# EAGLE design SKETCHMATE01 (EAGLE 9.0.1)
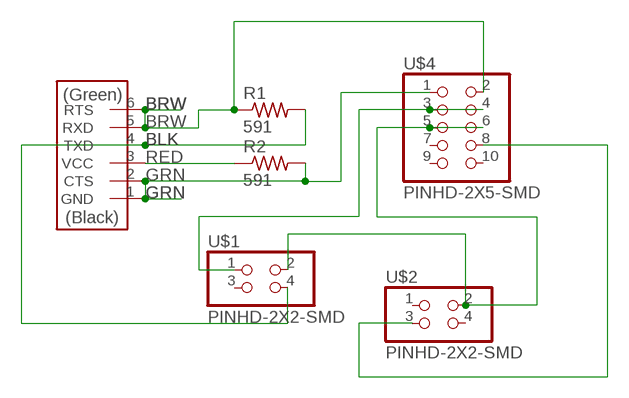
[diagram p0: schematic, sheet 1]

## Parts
R1  591  RES-US1206FAB  [R1206FAB]
R2  591  RES-US1206FAB  [R1206FAB]
U$1  PINHD-2X2-SMD  [2X02SMD]
U$2  PINHD-2X2-SMD  [2X02SMD]
U$4  PINHD-2X5-SMD  [2X05SMD]
YEL  FTDI-SMD-HEADER  [1X06SMD]

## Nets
BLK: R1.2 U$1.4 YEL.4(TXD)
BRW: R1.1 U$4.2 YEL.5(RXD) YEL.6(RTS)
GRN: R2.2 U$4.1 YEL.1(GND) YEL.2(CTS)
N$1: U$1.1 U$4.3 U$4.4
N$2: U$1.2 U$2.2 U$4.5 U$4.6
N$3: U$2.3 U$4.8
RED: R2.1 YEL.3(VCC)
Unconnected: U$1.3 U$2.1 U$2.4 U$4.7 U$4.9 U$4.10

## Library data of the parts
R1 R2 = fablibrary:RES-US: Resistor (US Symbol)
U$1 U$2 = fablibrary:PINHD-2X2-SMD
U$4 = fablibrary:PINHD-2X5-SMD
YEL = fablibrary:FTDI-SMD-HEADER

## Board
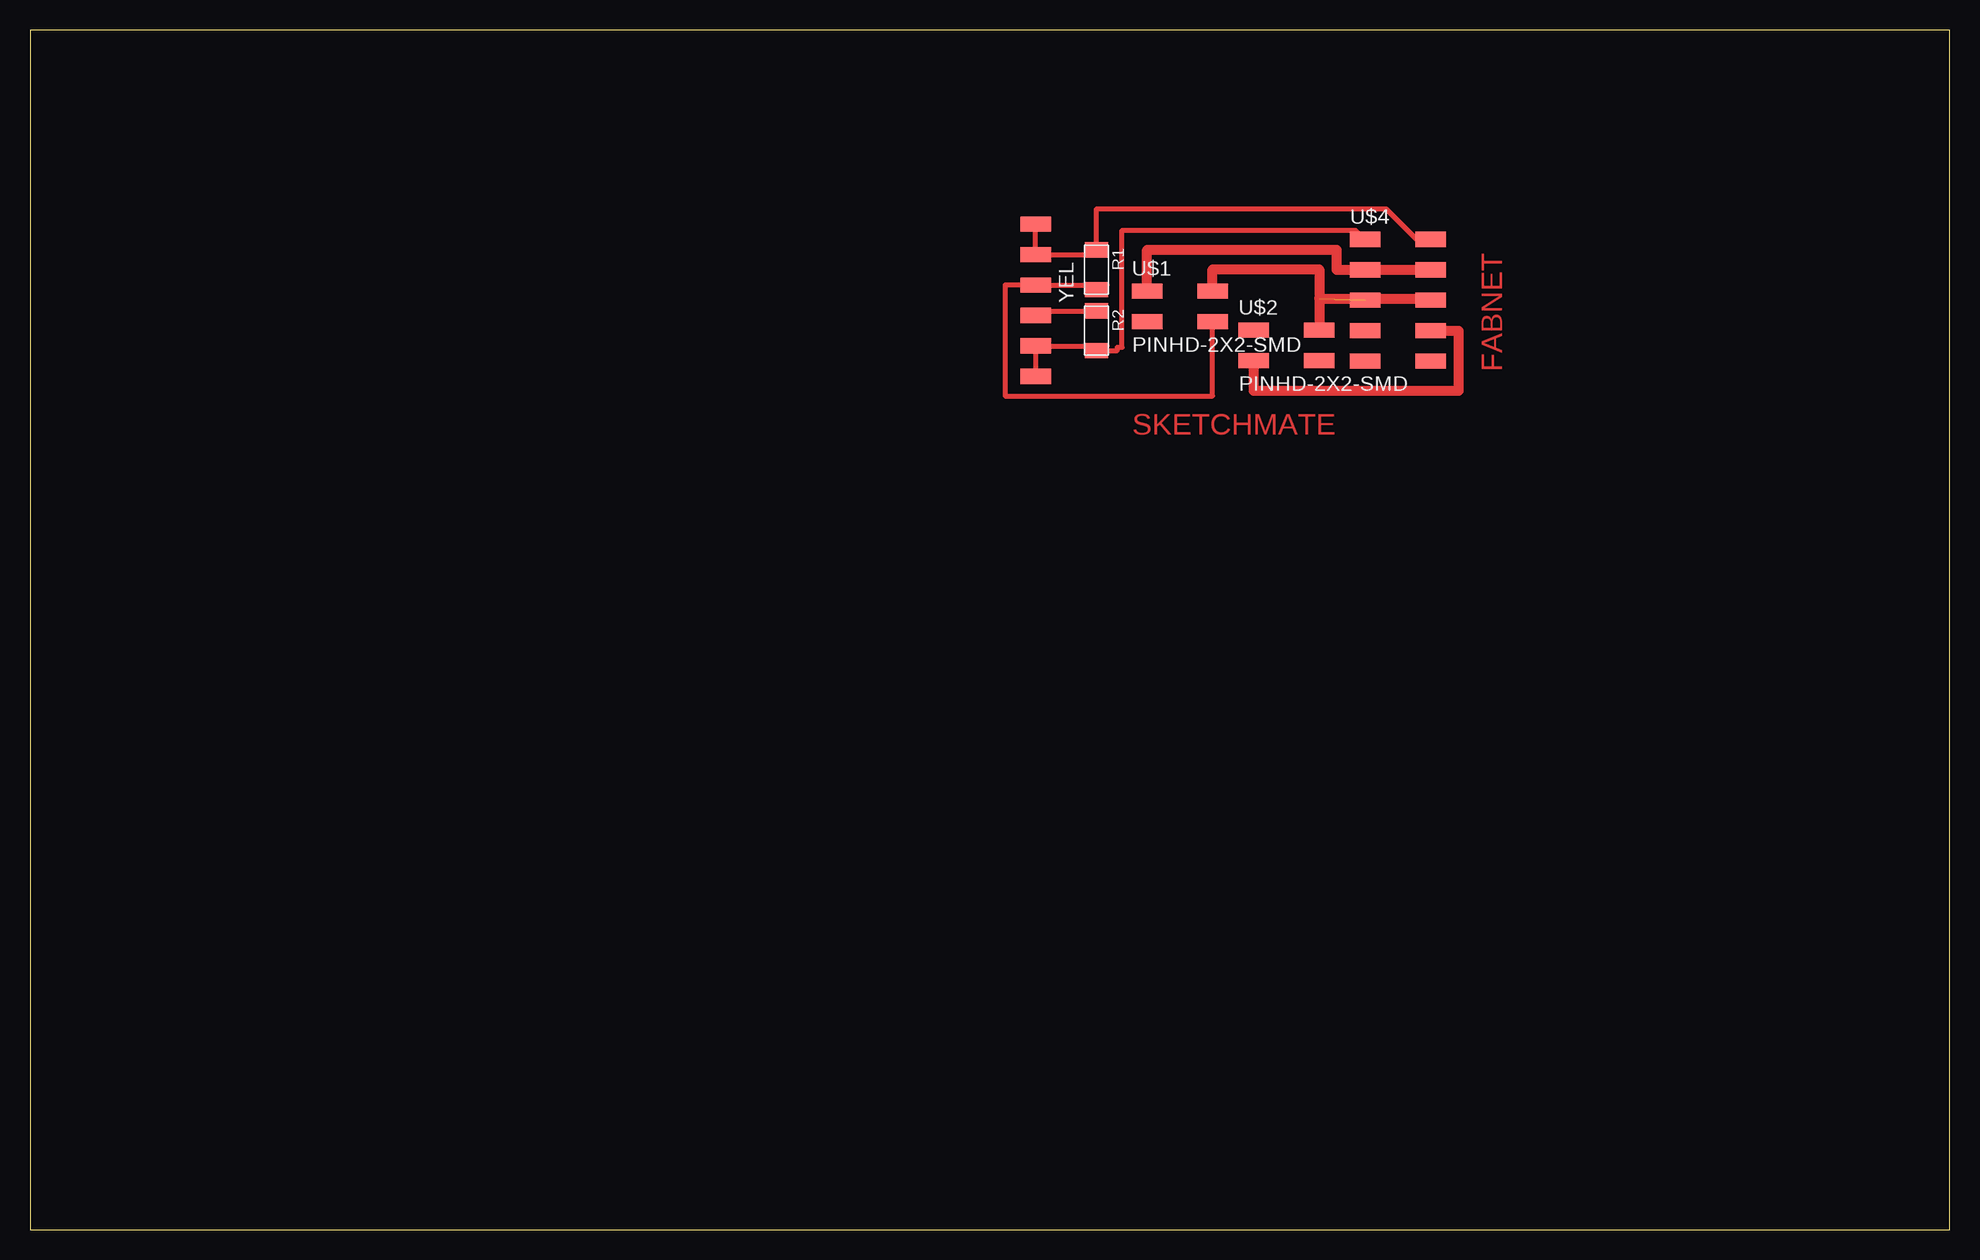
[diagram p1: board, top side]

Size 160 x 100 mm. Coordinates in mm from the lower left corner, seen from the top.
Outline: 0,0 160,0 160,100 0,100 0,0
Copper layers (1*16): Top 0.035mm / dielectric 1.5mm / Bottom 0.035mm
Design rules "default": minimum track width 6mil, minimum drill 0.35mm, track to track 6mil, track to pad 6mil, pad to pad 6mil, via to via 6mil, smd to smd 6mil, copper to edge 40mil, drill to drill 6mil, minimum pad ring 10mil, minimum via ring 8mil, stop-mask expansion 4mil, vias tented up to drill 0mil, thermal gap 10mil

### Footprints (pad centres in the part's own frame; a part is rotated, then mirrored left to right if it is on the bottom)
R1206FAB = smd 1.27 x 1.905: 1 -1.651,0; 2 1.651,0
2X02SMD = smd 2.54 x 1.27: 1 -2.54,1.27; 2 2.92,1.27; 3 -2.54,-1.27; 4 2.92,-1.27
2X05SMD = smd 2.54 x 1.27: 1 -2.54,2.54; 2 2.92,2.54; 3 -2.54,0; 4 2.92,0; 5 -2.54,-2.54; 6 2.92,-2.54; 7 -2.54,-5.08; 8 2.92,-5.08; 9 -2.54,-7.62; 10 2.92,-7.62
1X06SMD = smd 2.54 x 1.27: 1 0,6.35; 2 0,3.81; 3 0,1.27; 4 0,-1.27; 5 0,-3.81; 6 0,-6.35

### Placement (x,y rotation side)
R1  88.9,80.01 270 top
R2  88.9,74.93 270 top
U$1  95.66,76.96 0 top
U$2  104.55,73.71 0 top
U$4  113.84,80.01 0 top
YEL  83.82,77.47 180 top

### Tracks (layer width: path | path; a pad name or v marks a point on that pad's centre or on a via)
BLK
  Top 0.406: R1.2 89.79,78.74 YEL.4 81.28,78.74 81.28,69.49 98.58,69.49 U$1.4
BRW
  Top 0.406: 115.95,82.93 U$4.2 115.57,82.55 113.03,85.09 88.9,85.09 R1.1 88.9,81.28 YEL.5 YEL.6
GRN
  Top 0.406: U$4.1 110.49,83.31 91.03,83.31 91.03,73.56 90.63,73.56 90.63,73.28 R2.2 89.79,73.66 YEL.2 YEL.1
N$1
  Top 0.813: U$4.4 U$4.3 108.92,80.01 108.92,81.69 93.12,81.69 U$1.1
N$2  (1 unrouted)
  Top 0.813: U$1.2 98.58,80.06 107.47,80.06 107.47,77.62 | 107.47,77.62 U$2.2 | 107.47,77.62 116.76,77.62 U$4.6
N$3
  Top 0.813: U$4.8 119.08,74.93 119.08,69.9 102.01,69.9 U$2.3
RED
  Top 0.406: YEL.3 84.2,76.58 R2.1

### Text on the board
Top: FABNET | SKETCHMATE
